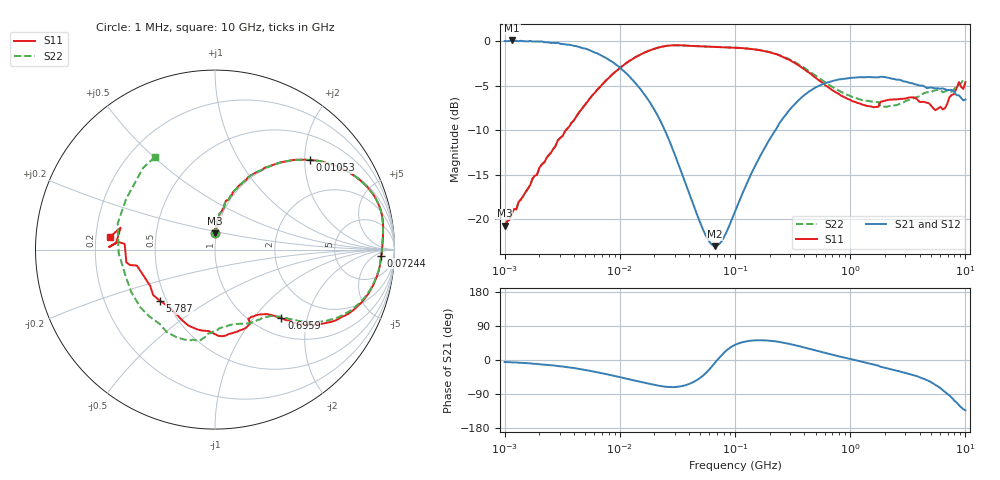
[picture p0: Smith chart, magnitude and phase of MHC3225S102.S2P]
!Agilent Technologies,E5071C,MY46111244,A.11.31
!Date: Thu May 09 18:29:32 2019
!Data & Calibration Information:
!Freq	S11:SOLT2(ON)	S21:SOLT2(ON)	S12:SOLT2(ON)	S22:SOLT2(ON)
# Hz S dB R 50
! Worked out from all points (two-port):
!   201 points, 1 MHz to 10 GHz, reference 50 ohm
!   highest |S21| = 0.09 dB at 1.159 MHz (marker M1); lowest = -23.0 dB at 66.4 MHz (marker M2)
!   |S21| within 3 dB of the highest: start of sweep to 9.923 MHz
!   lowest |S11| = -20.7 dB at 1 MHz (marker M3), VSWR 1.20, Z = 49.3 + j9.14 ohm
!   |S11| at or under -10 dB: start of sweep to 3.408 MHz
!   |S22| runs from -20.8 to -0.5 dB; largest |S21 - S12| = 0.0087
!   S11 on the Smith chart (normalised r, x): 1 MHz: 0.99, +0.18; 10.53 MHz: 1.00, +2.11; 72.44 MHz: 22, -10; 695.9 MHz: 1.32, -1.41; 5.787 GHz: 0.46, -0.32; 10 GHz: 0.26, +0.06
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1000000  -20.74 89.0  0.02 -5.4  -0.00 -5.3  -20.76 88.5
1159128  -19.29 91.7  0.09 -6.2  0.07 -6.0  -19.36 92.1
4810209  -7.41 65.9  -0.79 -25.4  -0.77 -25.3  -7.41 66.1
1.053043e7  -2.78 43.4  -3.22 -46.8  -3.22 -46.8  -2.79 43.5
2.206931e7  -0.68 20.9  -8.73 -68.1  -8.75 -68.1  -0.68 21.1
6.639937e7  -0.64 -0.9  -23.04 -8.7  -23.03 -8.6  -0.64 -0.6
7.24436e7  -0.66 -2.1  -22.85 4.6  -22.85 4.6  -0.66 -1.6
1.047129e8  -0.73 -7.6  -18.52 42.6  -18.52 42.5  -0.73 -7.0
2.418599e8  -1.59 -24.6  -9.26 47.5  -9.26 47.5  -1.55 -23.2
4.810209e8  -3.94 -40.6  -5.34 26.7  -5.35 26.7  -3.71 -38.0
6.959176e8  -5.48 -45.9  -4.48 14.1  -4.49 14.1  -5.13 -43.6
1.59878e9  -7.42 -61.7  -4.05 -11.8  -4.05 -11.9  -6.75 -60.5
2.206931e9  -6.57 -69.0  -4.14 -23.7  -4.13 -23.7  -7.27 -81.7
3.630781e9  -6.35 -87.6  -4.83 -41.0  -4.84 -40.9  -6.35 -95.7
4.83488e9  -6.98 -109.6  -5.22 -55.6  -5.22 -55.6  -5.73 -102.5
5.786901e9  -7.57 -137.0  -5.29 -69.8  -5.35 -69.8  -5.46 -113.3
6.952868e9  -7.05 -168.4  -5.50 -88.9  -5.48 -89.0  -5.59 -142.1
7.585776e9  -6.04 -171.8  -5.47 -98.7  -5.46 -98.7  -5.68 -164.3
7.988146e9  -5.95 176.4  -5.69 -106.8  -5.68 -106.7  -5.40 -178.2
8.792888e9  -4.58 178.6  -6.09 -119.0  -6.14 -118.7  -4.89 150.4
9.597629e9  -5.36 166.9  -6.66 -129.8  -6.66 -129.6  -4.35 131.4
1e10  -4.60 173.1  -6.54 -132.8  -6.53 -132.5  -4.21 122.8
